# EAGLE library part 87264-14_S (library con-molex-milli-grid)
RECEPTACAL
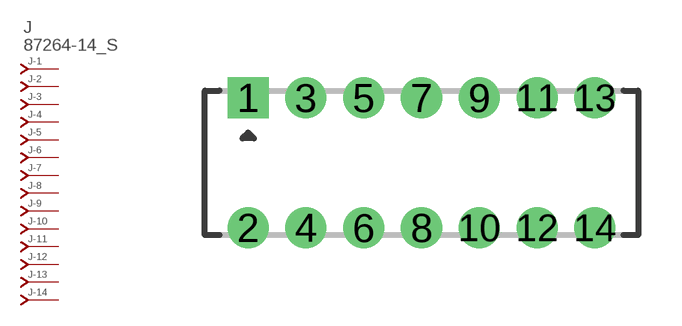
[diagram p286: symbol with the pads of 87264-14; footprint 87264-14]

Designator prefix J; gates -1=J-NV -2=J-N -3=J-N -4=J-N -5=J-N -6=J-N -7=J-N -8=J-N -9=J-N -10=J-N -11=J-N -12=J-N -13=J-N -14=J-N

## 87264-14_S  [87264-14]
1  -1:J  pas
2  -2:J  pas
3  -3:J  pas
4  -4:J  pas
5  -5:J  pas
6  -6:J  pas
7  -7:J  pas
8  -8:J  pas
9  -9:J  pas
10  -10:J  pas
11  -11:J  pas
12  -12:J  pas
13  -13:J  pas
14  -14:J  pas

## Footprint 87264-14 (pad centres in mm)
RECEPTACAL Dual Row, Side Entry
drill 0.914 square: 1 -6,2.25
drill 0.914: 2 -6,-2.25; 3 -4,2.25; 4 -4,-2.25; 5 -2,2.25; 6 -2,-2.25; 7 0,2.25; 8 0,-2.25; 9 2,2.25; 10 2,-2.25; 11 4,2.25; 12 4,-2.25; 13 6,2.25; 14 6,-2.25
